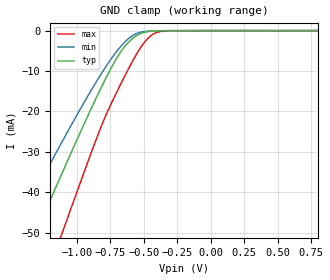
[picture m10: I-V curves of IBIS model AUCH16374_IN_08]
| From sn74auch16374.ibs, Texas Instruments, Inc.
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[Model]   AUCH16374_IN_08
Model_type  Input
Vinl=0
Vinh=0.8
| variable   typ   min   max
C_comp   2.85pF   2.40pF   3.21pF
[Temperature Range]   40   100   -40
| Ambient temperature   25   85   -40
[Voltage range]   0.8   0.8   0.8
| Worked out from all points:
|   GND clamp passes 1 mA (typ) near -0.54 V on its own axis
[GND Clamp]
| AUCH16374_IN_08
|   Voltage   I(typ)   I(min)   I(max)
-3.6V     -229mA     -190.7mA   -276.9mA
-1.495V   -64.59mA   -51.38mA   -85.52mA
-1.45V    -61.11mA   -48.52mA   -81.37mA
-1.32V    -51.11mA   -40.33mA   -69.38mA
-1.275V   -47.66mA   -37.53mA   -65.23mA
-1.115V   -35.54mA   -27.71mA   -50.46mA
-825mV    -14.49mA   -11.02mA   -24.24mA
-695mV    -6.395mA   -4.788mA   -14.7mA
-580mV    -1.846mA   -1.16mA    -7.304mA
-450mV    -162.3uA   -82.69uA   -1.323mA
-305mV    -21.19uA   -13.94uA   -49.01uA
800mV     109.4pA    198.3pA    88.89pA
